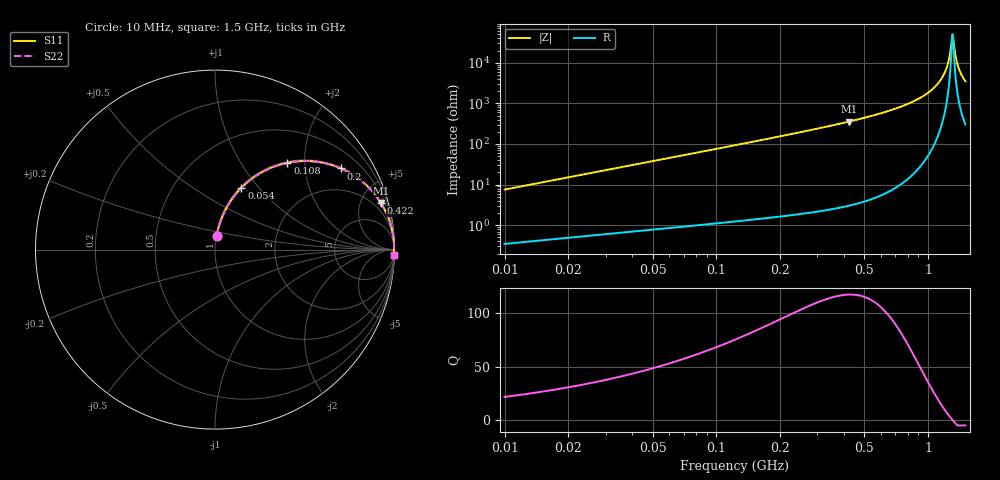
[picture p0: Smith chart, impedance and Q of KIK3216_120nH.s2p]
!version-2
!date-01.2022
!Series
# MHz S RI R 50
!Freq ReS11 ImS11 ReS21 ImS21 ReS12 ImS12 ReS22 ImS22
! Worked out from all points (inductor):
!   746 points, 10 MHz to 1.5 GHz, reference 50 ohm
!   read as one part in series: L = 120 nH near 16 MHz
!   highest Q = 118 at 422 MHz (marker M1), where L = 134 nH
!   self-resonance near 1.304 GHz
!   S11 on the Smith chart (normalised r, x): 10 MHz: 1.01, +0.15; 54 MHz: 1.02, +0.82; 108 MHz: 1.02, +1.64; 200 MHz: 1.03, +3.09; 422 MHz: 1.06, +7.11; 1.5 GHz: 7, -70
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10  0.00905 0.0745  0.991 -0.0745  0.991 -0.0745  0.00905 0.0745
30  0.0539 0.2128  0.9461 -0.2128  0.9461 -0.2128  0.0539 0.2128
54  0.1475 0.3449  0.8525 -0.3449  0.8525 -0.3449  0.1475 0.3449
78  0.2618 0.4315  0.7382 -0.4315  0.7382 -0.4315  0.2618 0.4315
108  0.4034 0.4836  0.5966 -0.4836  0.5966 -0.4836  0.4034 0.4836
200  0.7026 0.4518  0.2974 -0.4518  0.2974 -0.4518  0.7026 0.4518
260  0.8042 0.3921  0.1958 -0.3921  0.1958 -0.3921  0.8042 0.3921
422  0.9247 0.2596  0.0753 -0.2596  0.0753 -0.2596  0.9247 0.2596
508  0.9516 0.2104  0.0484 -0.2104  0.0484 -0.2104  0.9516 0.2104
756  0.9852 0.1147  0.0148 -0.1147  0.0148 -0.1147  0.9852 0.1147
1004  0.9956 0.0536  0.00443 -0.0536  0.00443 -0.0536  0.9956 0.0536
1162  0.9977 0.0236  0.0023 -0.0236  0.0023 -0.0236  0.9977 0.0236
1214  0.998 0.0147  0.00205 -0.0147  0.00205 -0.0147  0.998 0.0147
1252  0.998 0.00842  0.00197 -0.00842  0.00197 -0.00842  0.998 0.00842
1274  0.998 0.00489  0.00196 -0.00489  0.00196 -0.00489  0.998 0.00489
1298  0.998 0.00112  0.00199 -0.00112  0.00199 -0.00112  0.998 0.00112
1306  0.998 -0.000128  0.002 0.000128  0.002 0.000128  0.998 -0.000128
1312  0.998 -0.00106  0.00201 0.00106  0.00201 0.00106  0.998 -0.00106
1342  0.9979 -0.00563  0.00211 0.00563  0.00211 0.00563  0.9979 -0.00563
1376  0.9977 -0.0107  0.00226 0.0107  0.00226 0.0107  0.9977 -0.0107
1430  0.9974 -0.0185  0.00261 0.0185  0.00261 0.0185  0.9974 -0.0185
1500  0.9968 -0.0282  0.00323 0.0282  0.00323 0.0282  0.9968 -0.0282
